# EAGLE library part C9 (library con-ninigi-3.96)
NINIGI
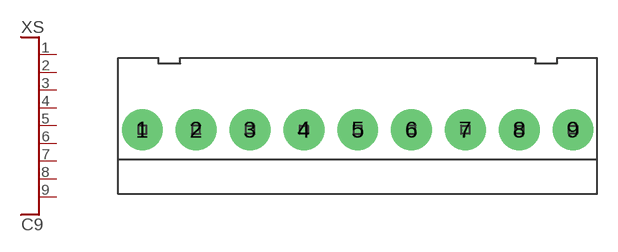
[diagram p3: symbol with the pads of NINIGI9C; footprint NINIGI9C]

Designator prefix XS

## C9  [NINIGI9C]
1  P$1
2  P$2
3  P$3
4  P$4
5  P$5
6  P$6
7  P$7
8  P$8
9  P$9

## Footprint NINIGI9C (pad centres in mm)
drill 1.6 pad 3: 1 -15.84,0; 2 -11.88,0; 3 -7.92,0; 4 -3.96,0; 5 0,0; 6 3.96,0; 7 7.92,0; 8 11.88,0; 9 15.84,0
